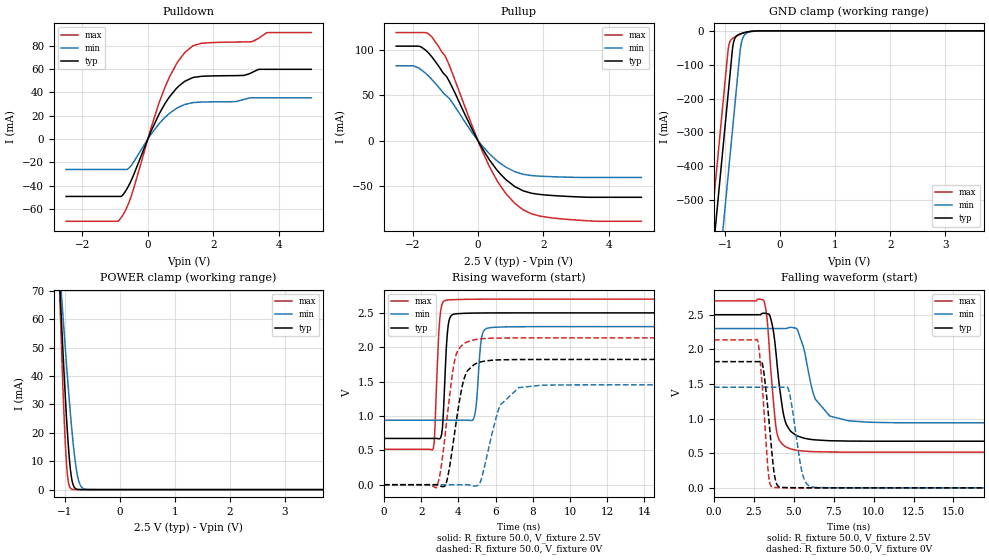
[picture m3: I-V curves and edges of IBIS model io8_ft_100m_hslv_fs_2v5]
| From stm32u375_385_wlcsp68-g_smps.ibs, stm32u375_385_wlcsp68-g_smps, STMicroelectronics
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[Model]   io8_ft_100m_hslv_fs_2v5
Model_type I/O
Polarity   Non-Inverting
Enable   Active-Low
| CAP_THRESHOLD on pad IOFT is "UDTCAPC" :
| Rising=30.0% of vddiom   Falling=70.0% of vddiom
| C_comp min and max val. don't necessarily correlate with the min and max pvt
| but are the smallest and greatest pad capacitance found.
| var   typ   min   max
C_comp   3.68195pF  3.67098pF  3.72549pF
|C_comp_pullup   2.08707pF  2.19349pF  2.32533pF
|C_comp_pulldown   1.59489pF  1.47749pF  1.40017pF
Vinl = 1.15V
Vinh = 1.35V
Vmeas = 1.25V   | Reference voltage for timing measurements
Cref  = 50.0pF   | Timing specification test load capacitance value
Rref  = 1.0MOhm   | Timing specification test load resistance value
Vref  = 1.375V   | Timing specification test load voltage
[Model Spec]
| TIME_THRESHOLD on pin ZIV11 is "CMOS" :
| Rising=50.0% of vdd   Falling=50.0% of vdd
Vinl 981.50000mV 911.50000mV 1.04650V
Vinh 1.42350V 1.31650V 1.50350V
| variable   typ   min   max
[Temperature Range] 25.0 130.0 -40.0
| variable   typ   min   max
[Voltage Range] 2.5V 2.3V 2.7V
| variable   typ   min   max
[POWER Clamp Reference] 2.5V 2.3V 2.7V
| variable   typ   min   max
[GND Clamp Reference] 0V 0V 0V
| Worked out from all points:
|   slope of the pulldown table from 0 to 0.375 V, typ, clamps not added: 16.4 ohm
|   slope of the pullup table from 0 to 0.375 V, typ, clamps not added: 16.7 ohm
|   GND clamp passes 1 mA (typ) near -0.50 V on its own axis
|   POWER clamp passes 1 mA (typ) near -0.83 V on its own axis
|   rising waveform, R_fixture 50.0, V_fixture 2.5V: 20-80 % time 197ps typ, 217ps min, 201ps max; typ from 0.673 V to 2.5 V
|   falling waveform, R_fixture 50.0, V_fixture 2.5V: 20-80 % time 581ps typ, 999ps min, 454ps max; typ from 2.5 V to 0.673 V
|   rising waveform, R_fixture 50.0, V_fixture 0V: 20-80 % time 637ps typ, 835ps min, 576ps max; typ from 0 V to 1.82 V
|   falling waveform, R_fixture 50.0, V_fixture 0V: 20-80 % time 460ps typ, 565ps min, 392ps max; typ from 1.82 V to 0 V
[POWER Clamp]
-2.5V     736.6mA    513.9mA    1.064A
-1.1V     75.38mA    79.63mA    73.18mA
-1.09V    71.2mA     76.8mA     67.14mA
-1.08V    67.05mA    73.98mA    61.2mA
-1.06V    58.89mA    68.38mA    49.67mA
-1.02V    43.22mA    57.4mA     28.67mA
-980mV    28.81mA    46.77mA    12.28mA
-940mV    16.45mA    36.61mA    3.257mA
-880mV    4.35mA     22.67mA    225.4uA
-770mV    97.5uA     4.87mA     1.193uA
-630mV    518.5nA    149.1uA    1.636nA
5V        0A         0A         0A
[GND Clamp]
-2.5V     -2.831A    -3.071A    -2.699A
-1.46V    -1.063A    -1.303A    -931.1mA
-1.21V    -637.8mA   -878.3mA   -506.1mA
-950mV    -195.8mA   -436.3mA   -64.07mA
-940mV    -178.8mA   -419.3mA   -50.67mA
-910mV    -127.8mA   -368.3mA   -31.36mA
-850mV    -37.25mA   -266.3mA   -20.72mA
-750mV    -10.68mA   -96.33mA   -12.3mA
-710mV    -8.126mA   -41.01mA   -9.515mA
-670mV    -6.142mA   -18.5mA    -7.051mA
-470mV    -612.4uA   -1.154mA   -431uA
5V        1.687nA    211.8nA    737.8pA
| variable   typ   min   max
[Pullup Reference] 2.5V 2.3V 2.7V
| variable   typ   min   max
[Pulldown Reference] 0V 0V 0V
[Pullup]
-2.5V     103.9mA    82.33mA    118.9mA
-1.98V    103.9mA    82.23mA    118.9mA
-1.74V    103mA      78.1mA     118.9mA
-1.5V     95.96mA    70.63mA    117.1mA
-1.21V    82.39mA    59.12mA    104mA
-890mV    66.01mA    46.86mA    84.06mA
-170mV    11.87mA    8.299mA    15.68mA
350mV     -21.19mA   -14.53mA   -28.53mA
850mV     -42.77mA   -29.12mA   -58.03mA
1.38V     -55.27mA   -37.08mA   -76.15mA
2.5V      -60.98mA   -40.04mA   -86.01mA
5V        -62.43mA   -40.58mA   -88.86mA
[Pulldown]
-2.5V     -49.09mA   -26.02mA   -70.37mA
-920mV    -49.09mA   -26.02mA   -70.37mA
-830mV    -49.09mA   -26.02mA   -67.8mA
-510mV    -35.57mA   -22.69mA   -49.05mA
90mV      6.138mA    3.798mA    8.848mA
520mV     30.1mA     18.41mA    43.96mA
940mV     45.18mA    27.25mA    67.1mA
1.38V     52.7mA     31.24mA    79.88mA
2.68V     54.32mA    32.09mA    83.06mA
3.2V      57.2mA     35.33mA    83.52mA
3.67V     59.71mA    35.33mA    91.16mA
5V        59.71mA    35.33mA    91.17mA
[Ramp]
dV/dt_r 1.09344V/636.18597ps 871.78284mV/823.14442ps 1.28161V/575.20435ps
dV/dt_f 1.09609V/578.71489ps 816.99021mV/880.56958ps 1.31053V/452.20659ps
R_load = 50.0
| Removed startup time: 0s 0s 0s  .
| Removed end time: 19.25ns.
[Rising Waveform]
R_fixture   = 50.0
V_fixture   = 2.5V
V_fixture_min = 2.3V
V_fixture_max = 2.7V
0s        673.2mV    938.3mV    515.8mV
2.65ns    673.2mV    938.3mV    527.1mV
3ns       668.4mV    938.4mV    2.406V
3.25ns    1.368V     938.3mV    2.676V
3.4ns     2.175V     938.4mV    2.686V
3.55ns    2.43V      938.4mV    2.69V
4.85ns    2.497V     981.6mV    2.698V
5.25ns    2.498V     2.139V     2.699V
5.55ns    2.499V     2.276V     2.699V
19.25ns   2.5V       2.3V       2.7V
| Removed startup time: 0s 0s 0s  .
| Removed end time: 59.25ns.
[Falling Waveform]
R_fixture   = 50.0
V_fixture   = 2.5V
V_fixture_min = 2.3V
V_fixture_max = 2.7V
0s        2.5V       2.3V       2.7V
3.1ns     2.522V     2.3V       2.71V
3.3ns     2.516V     2.3V       2.485V
3.55ns    2.444V     2.3V       1.713V
3.95ns    1.782V     2.3V       784mV
4.45ns    968.4mV    2.299V     599mV
5.2ns     752.3mV    2.289V     541.7mV
6.35ns    692.4mV    1.279V     521.9mV
8.45ns    675.3mV    967.5mV    516.4mV
59.25ns   673.2mV    938.3mV    515.8mV
| Removed startup time: 0s 0s 0s  .
| Removed end time: 59.25ns.
[Rising Waveform]
R_fixture   = 50.0
V_fixture   = 0V
V_fixture_min = 0V
V_fixture_max = 0V
0s        5.238nV    85.5nV     4.322nV
2.85ns    -168.3uV   -218.5nV   -26.27mV
3.35ns    23.57mV    -4.577uV   867mV
3.85ns    849.1mV    -15.72uV   1.865V
4.35ns    1.575V     -127.8uV   2.06V
5.05ns    1.774V     -10mV      2.118V
6.25ns    1.817V     1.159V     2.134V
7.25ns    1.821V     1.413V     2.135V
8.45ns    1.822V     1.447V     2.136V
59.25ns   1.822V     1.453V     2.136V
| Removed startup time: 0s 0s 0s  .
| Removed end time: 19.25ns.
[Falling Waveform]
R_fixture   = 50.0
V_fixture   = 0V
V_fixture_min = 0V
V_fixture_max = 0V
0s        1.822V     1.453V     2.136V
2.7ns     1.823V     1.453V     2.142V
3.1ns     1.702V     1.453V     1.212V
3.4ns     1.071V     1.453V     211.1mV
3.65ns    447.1mV    1.453V     11.36mV
3.95ns    44.54mV    1.453V     3.979mV
4.65ns    3.32mV     1.432V     1.929mV
5.5ns     1.449mV    238.8mV    897.3uV
5.95ns    973.5uV    28.84mV    605.7uV
19.25ns   5.179uV    19.17uV    1.585uV
